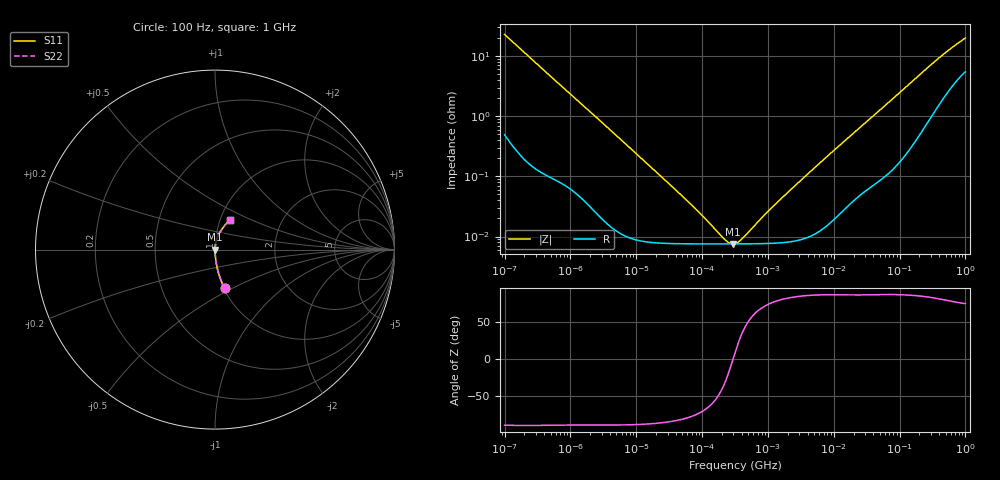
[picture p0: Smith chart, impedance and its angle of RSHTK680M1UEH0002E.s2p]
! RSHTK680M1UEH0002E  S-PARAMETER MODEL  (General Type)
! Model Generated by ELNA Corporation (http://www.ty-top.com)
! Version 1.0
! ELNA Control No. 201216
! Copyright (c) 2020 ELNA CO.,LTD. All Rights Reserved.
! Products Name : CONDUCTIVE POLYMER HYBRID ALUMINUM ELECTROLYTIC CAPACITORS
! Characteristics :
!  Capacitance  :  68uF  ,  Rated voltage  :  50V
!  Operating Temp. Range  :  -55 to +125 degC  ,  Endurance  :  4000hr at 125 degC
!  Dimension D  :  8mm  ,  Dimension L  :  10mm
! Frequency Range : 100Hz - 1GHz
! External Node Assignments :
!  1  o---| |---o  2
# MHz S RI R 50
!Freq[MHz].  S11 Real  S11 Imag  S21 Real  S21 Imag  S12 Real  S12 Imag  S22 Real  S22 Imag
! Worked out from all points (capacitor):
!   401 points, 100 Hz to 1 GHz, reference 50 ohm
!   read as one part in series: C = 69.6 uF near 108 Hz
!   lowest |Z| = 7.53 mohm at 291.7 kHz (marker M1)
!   series resonance near 295.6 kHz, so ESL is about 4.2 nH
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0.0001  0.0539 -0.2153  0.9461 0.2153  0.9461 0.2153  0.0539 -0.2153
0.000113  0.043 -0.1931  0.957 0.1931  0.957 0.1931  0.043 -0.1931
0.000183  0.0174 -0.1226  0.9826 0.1226  0.9826 0.1226  0.0174 -0.1226
0.000309  0.00674 -0.0736  0.9933 0.0736  0.9933 0.0736  0.00674 -0.0736
0.000613  0.00226 -0.0375  0.9977 0.0375  0.9977 0.0375  0.00226 -0.0375
0.001488  0.000675 -0.0158  0.9993 0.0158  0.9993 0.0158  0.000675 -0.0158
0.022131  7.89e-05 -0.00107  0.9999 0.00107  0.9999 0.00107  7.89e-05 -0.00107
0.080353  7.54e-05 -0.000275  0.9999 0.000275  0.9999 0.000275  7.54e-05 -0.000275
0.187284  7.53e-05 -7.63e-05  0.9999 7.63e-05  0.9999 7.63e-05  7.53e-05 -7.63e-05
0.211349  7.53e-05 -5.52e-05  0.9999 5.52e-05  0.9999 5.52e-05  7.53e-05 -5.52e-05
0.291743  7.53e-05 -2.11e-06  0.9999 2.11e-06  0.9999 2.11e-06  7.53e-05 -2.11e-06
0.316228  7.53e-05 1.09e-05  0.9999 -1.09e-05  0.9999 -1.09e-05  7.53e-05 1.09e-05
0.419276  7.54e-05 5.76e-05  0.9999 -5.76e-05  0.9999 -5.76e-05  7.54e-05 5.76e-05
0.473151  7.55e-05 7.88e-05  0.9999 -7.88e-05  0.9999 -7.88e-05  7.55e-05 7.88e-05
0.767361  7.6e-05 0.000179  0.9999 -0.000179  0.9999 -0.000179  7.6e-05 0.000179
1.148154  7.7e-05 0.000293  0.9999 -0.000293  0.9999 -0.000293  7.7e-05 0.000293
4.704354  0.000106 0.00127  0.9999 -0.00127  0.9999 -0.00127  0.000106 0.00127
69.9842  0.00145 0.0173  0.9986 -0.0173  0.9986 -0.0173  0.00145 0.0173
176.8072  0.00575 0.0426  0.9943 -0.0426  0.9943 -0.0426  0.00575 0.0426
380.1894  0.0215 0.0852  0.9785 -0.0852  0.9785 -0.0852  0.0215 0.0852
668.3439  0.0509 0.1304  0.9491 -0.1304  0.9491 -0.1304  0.0509 0.1304
1000  0.0823 0.1669  0.9177 -0.1669  0.9177 -0.1669  0.0823 0.1669
